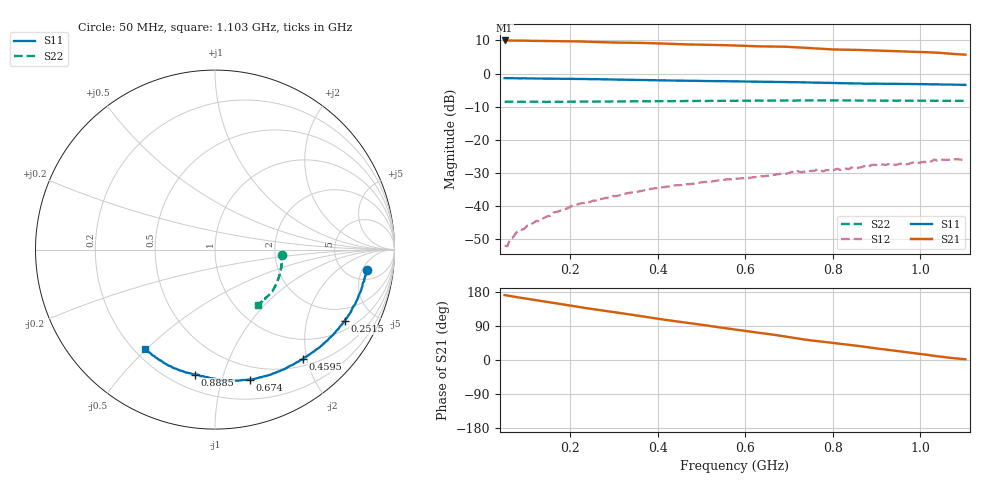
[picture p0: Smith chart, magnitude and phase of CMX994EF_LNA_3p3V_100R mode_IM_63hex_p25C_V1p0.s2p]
! CMX994EF, LNA s-parameters at Vcc = 3.3V, 100R mode, IM reg = 63hex, de-embedded to DUT
! Created: GMT 2025-09-22 10:51:28
# Hz S MA R 50
! freq[Hz]  S11[mag]  S11[ang]  S21[mag]  S21[ang]  S12[mag]  S12[ang]  S22[mag]  S22[ang]
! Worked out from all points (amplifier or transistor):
!   163 points, 50 MHz to 1.103 GHz, reference 50 ohm
!   highest |S21| = 10.0 dB at 50 MHz (marker M1)
!   |S21| within 3 dB of that: start of sweep to 889.3 MHz
!   unconditionally stable (mu >= 1): start of sweep to end of sweep
!   at 225.5 MHz: K = 4.08, MAG = 15.3 dB, |S12| = -39.1 dB
!   at 576.5 MHz: K = 2.78, MAG = 12.8 dB, |S12| = -31.7 dB
!   at 1.103 GHz: K = 2.55, MAG = 8.8 dB, |S12| = -25.7 dB
!   S11 on the Smith chart (normalised r, x): 50 MHz: 7.56, -6.27; 251.5 MHz: 1.35, -3.37; 459.5 MHz: 0.61, -1.92; 674 MHz: 0.37, -1.23; 888.5 MHz: 0.29, -0.81; 1.103 GHz: 0.24, -0.50
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5e7  0.8552 -7.5  3.159 171.3  0.002537 88.6  0.3772 -4.5
5.65e7  0.8536 -8.0  3.153 170.0  0.0025 87.9  0.3767 -4.5
6.3e7  0.8519 -8.7  3.151 168.6  0.003221 87.7  0.3769 -4.6
8.25e7  0.85 -10.6  3.139 165.0  0.004353 84.4  0.3754 -4.9
1.67e8  0.8392 -19.6  3.091 149.8  0.008164 82.9  0.3767 -7.3
2.255e8  0.8291 -26.0  3.047 138.9  0.0111 77.1  0.3769 -10.0
2.515e8  0.8244 -28.9  3.008 134.2  0.01213 75.2  0.3768 -11.0
3.425e8  0.8057 -38.8  2.916 119.1  0.01619 71.8  0.3813 -14.6
4.01e8  0.7924 -45.1  2.855 108.8  0.0187 69.2  0.3838 -17.0
4.595e8  0.7814 -51.4  2.763 99.3  0.02095 66.8  0.3854 -19.5
5.31e8  0.7708 -59.1  2.71 87.8  0.0241 63.8  0.388 -22.8
5.765e8  0.7646 -64.1  2.651 80.3  0.02606 61.6  0.388 -25.0
6.74e8  0.7498 -75.1  2.557 64.9  0.0302 59.9  0.3912 -30.2
7.13e8  0.7421 -79.3  2.505 58.0  0.03215 55.9  0.3913 -32.1
7.52e8  0.7325 -83.8  2.407 51.5  0.03403 55.6  0.3938 -34.2
8.365e8  0.7119 -93.4  2.285 40.3  0.03632 55.1  0.3941 -38.2
8.885e8  0.7051 -99.2  2.237 32.4  0.04188 50.8  0.3931 -40.9
9.275e8  0.7031 -103.9  2.191 26.6  0.04317 47.4  0.39 -43.3
1.025e9  0.6883 -115.9  2.087 12.0  0.04717 46.2  0.3903 -48.3
1.032e9  0.6889 -116.7  2.075 11.1  0.05084 47.2  0.3889 -48.5
1.064e9  0.6842 -120.4  2.009 6.3  0.05032 44.5  0.3889 -50.0
1.103e9  0.676 -125.0  1.93 2.0  0.05191 41.3  0.3897 -52.5
